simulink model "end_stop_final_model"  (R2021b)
settings: Solver=VariableStepAuto  StartTime=0.0  StopTime=20  RelTol=1e-3
libraries: fl_lib x16, nesl_utility x4, sdl_lib x1

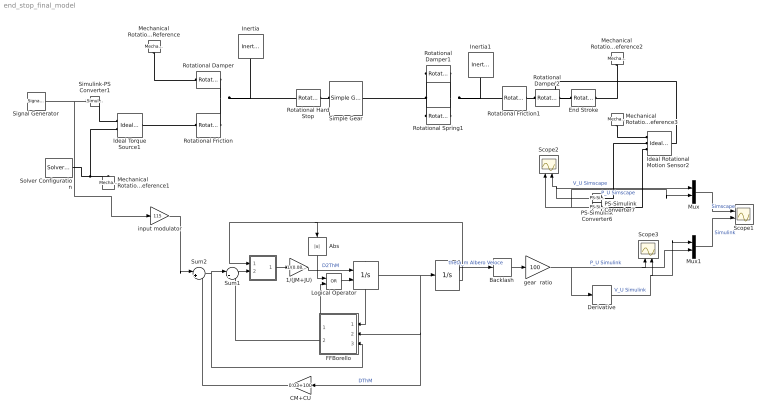
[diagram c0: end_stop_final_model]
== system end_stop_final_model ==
  " " : Integrator  ExternalReset=rising  ShowStatePort=on
  "  " : Integrator  LimitOutput=on  UpperSaturationLimit=0.1  LowerSaturationLimit=-0.1  ShowSaturationPort=on
  "                       " : Subsystem
  1/(JM+JU) : Gain  Gain=1/(0.085+50)
  Abs : Abs
  Backlash : Backlash  BacklashWidth=0.0174
  CM+CU : Gain  Gain=0.03+100
  Derivative : Derivative
  End Stroke : fl_lib/Mechanical/Rotational Elements/Rotational Hard Stop  upper_bnd=5 deg  lower_bnd=-5 deg  stiff_up=1e6 N*m/rad  stiff_low=1e6 N*m/rad  D_up=0.01 N*m/(rad/s)  D_low=0.01 N*m/(rad/s)  model=simscape.enum.hardstop.smooth  transition=0.001 rad  w_specify=off  w_priority=None  w=0 rad/s  w_nominal_specify=off  w_nominal_unit=rad/s  w_nominal_value=1  t_specify=off  t_priority=None  t=0 N*m  t_nominal_specify=off  t_nominal_unit=N*m  t_nominal_value=1  phi_specify=off  phi_priority=High  phi=0 rad  phi_nominal_specify=off  phi_nominal_unit=rad  phi_nominal_value=1
  FFBorello : Subsystem
  Ideal Rotational Motion Sensor2 : fl_lib/Mechanical/Mechanical Sensors/Ideal Rotational Motion Sensor  wrap_angle=simscape.enum.onoff.off  offset=0 rad
  Ideal Torque Source1 : fl_lib/Mechanical/Mechanical Sources/Ideal Torque Source
  Inertia : fl_lib/Mechanical/Rotational Elements/Inertia  inertia=0.085 kg*m^2  num_ports=foundation.enum.numPorts2.one  w_specify=off  w_priority=High  w=0 rad/s  w_nominal_specify=off  w_nominal_unit=rad/s  w_nominal_value=1  t_specify=off  t_priority=None  t=0 N*m  t_nominal_specify=off  t_nominal_unit=N*m  t_nominal_value=1
  Inertia1 : fl_lib/Mechanical/Rotational Elements/Inertia  inertia=50 kg*m^2  num_ports=foundation.enum.numPorts2.one  w_specify=off  w_priority=High  w=0 rad/s  w_nominal_specify=off  w_nominal_unit=rad/s  w_nominal_value=1  t_specify=off  t_priority=None  t=0 N*m  t_nominal_specify=off  t_nominal_unit=N*m  t_nominal_value=1
  Logical Operator : Logic  Operator=OR  AllPortsSameDT=off  OutDataTypeStr=boolean
  Mechanical Rotational Reference{,1..3} (4 alike) : fl_lib/Mechanical/Rotational Elements/Mechanical Rotational Reference
  Mux : Mux  Inputs=2
  Mux1 : Mux  Inputs=2
  PS-Simulink Converter6 : nesl_utility/PS-Simulink Converter  PhysicalDomain=network_engine_domain  SubClassName=ps_output  LeftPortType=input  RightPortType=output  PseudoPeriodic=off  Frequencies=[]  Unit=inherit  AffineConversion=off
  PS-Simulink Converter7 : nesl_utility/PS-Simulink Converter  PhysicalDomain=network_engine_domain  SubClassName=ps_output  LeftPortType=input  RightPortType=output  PseudoPeriodic=off  Frequencies=[]  Unit=inherit  AffineConversion=off
  Rotational Damper : fl_lib/Mechanical/Rotational Elements/Rotational Damper  D=0.03 N*m/(rad/s)  w_specify=off  w_priority=None  w=0 rad/s  w_nominal_specify=off  w_nominal_unit=rad/s  w_nominal_value=1  t_specify=off  t_priority=None  t=0 N*m  t_nominal_specify=off  t_nominal_unit=N*m  t_nominal_value=1
  Rotational Damper1 : fl_lib/Mechanical/Rotational Elements/Rotational Damper  D=50 N*m/(rad/s)  w_specify=off  w_priority=None  w=0 rad/s  w_nominal_specify=off  w_nominal_unit=rad/s  w_nominal_value=1  t_specify=off  t_priority=None  t=0 N*m  t_nominal_specify=off  t_nominal_unit=N*m  t_nominal_value=1
  Rotational Damper2 : fl_lib/Mechanical/Rotational Elements/Rotational Damper  D=100 N*m/(rad/s)  w_specify=off  w_priority=None  w=0 rad/s  w_nominal_specify=off  w_nominal_unit=rad/s  w_nominal_value=1  t_specify=off  t_priority=None  t=0 N*m  t_nominal_specify=off  t_nominal_unit=N*m  t_nominal_value=1
  Rotational Friction : fl_lib/Mechanical/Rotational Elements/Rotational Friction  brkwy_trq=5 N*m  brkwy_vel=0.1 rad/s  Col_trq=5 N*m  visc_coef=0 N*m/(rad/s)  w_specify=off  w_priority=None  w=0 rad/s  w_nominal_specify=off  w_nominal_unit=rad/s  w_nominal_value=1  t_specify=off  t_priority=None  t=0 N*m  t_nominal_specify=off  t_nominal_unit=N*m  t_nominal_value=1
  Rotational Friction1 : fl_lib/Mechanical/Rotational Elements/Rotational Friction  brkwy_trq=500 N*m  brkwy_vel=0.1 rad/s  Col_trq=500 N*m  visc_coef=0 N*m/(rad/s)  w_specify=off  w_priority=None  w=0 rad/s  w_nominal_specify=off  w_nominal_unit=rad/s  w_nominal_value=1  t_specify=off  t_priority=None  t=0 N*m  t_nominal_specify=off  t_nominal_unit=N*m  t_nominal_value=1
  Rotational Hard Stop : fl_lib/Mechanical/Rotational Elements/Rotational Hard Stop  upper_bnd=1 deg  lower_bnd=-1 deg  stiff_up=1e6 N*m/rad  stiff_low=1e6 N*m/rad  D_up=0.01 N*m/(rad/s)  D_low=0.01 N*m/(rad/s)  model=simscape.enum.hardstop.smooth  transition=0.001 rad  w_specify=off  w_priority=None  w=0 rad/s  w_nominal_specify=off  w_nominal_unit=rad/s  w_nominal_value=1  t_specify=off  t_priority=None  t=0 N*m  t_nominal_specify=off  t_nominal_unit=N*m  t_nominal_value=1  phi_specify=off  phi_priority=High  phi=0 rad  phi_nominal_specify=off  phi_nominal_unit=rad  phi_nominal_value=1
  Rotational Spring1 : fl_lib/Mechanical/Rotational Elements/Rotational Spring  spr_rate=50 N*m/rad  w_specify=off  w_priority=None  w=0 rad/s  w_nominal_specify=off  w_nominal_unit=rad/s  w_nominal_value=1  t_specify=off  t_priority=None  t=0 N*m  t_nominal_specify=off  t_nominal_unit=N*m  t_nominal_value=1  phi_specify=off  phi_priority=High  phi=0 rad  phi_nominal_specify=off  phi_nominal_unit=rad  phi_nominal_value=1
  Scope1 : Scope  NumInputPorts=2
  Scope2 : Scope  NumInputPorts=2
  Scope3 : Scope  NumInputPorts=2
  Signal Generator : SignalGenerator  Amplitude=5  Units=rad/sec
  Simple Gear : sdl_lib/Gears/Simple Gear  ratio=100  rotation_direction=sdl.enum.shaftOutputDirection.same  friction_model=sdl.enum.gear_efficiencies_load.off  T_noload=0.1 N*m  T_nom=5 N*m  efficiency_nom=0.8  efficiency=0.8  temperature_TLU=[280, 300, 320] K  load_TLU=[1, 5, 10] N*m  efficiency_TLU=[.95, .9, .85]  efficiency_TLU2=[.85, .8, .75; .95, .9, .85; .85, .8, .7]  w_thr=0.01 rad/s  pwr_thr=0.001 W  backlash_model=sdl.enum.backlashModel.Off  backlash_distance=1e-3 mm  x0=0 mm  r_base=0.1 m  hardstop_model=simscape.enum.hardstop.smooth  transition=1e-4 mm  backlash_stiffness=1e7 N/m  backlash_damping=1e6 N/(m/s)  e=0  v_tol=0.001 m/s  mu_visc=[0, 0] N*m/(rad/s)  enable_faults=simscape.enum.onoff.off  efficiency_fault=0.05  external_fault=simscape.enum.onoff.off  temporal_fault=simscape.enum.onoff.off  fault_time=5 s  fault_angles=pi / 12 rad  report_fault=simscape.enum.assert.action.none  thermal_mass=50 J/K  temperature_specify=off  temperature_priority=High  temperature=300 K  temperature_nominal_specify=off  temperature_nominal_unit=K  temperature_nominal_value=1
  Simulink-PS Converter1 : nesl_utility/Simulink-PS Converter  PhysicalDomain=network_engine_domain  SubClassName=ps_input  LeftPortType=input  RightPortType=output  PseudoPeriodic=off  Frequencies=[]  NoiseDistribution=none  NoiseParameters=[]  Unit=1  AffineConversion=off  FilteringAndDerivatives=provide  SimscapeFilterOrder=1  InputFilterTimeConstant=0.001  UdotUserProvided=0
  Solver Configuration : nesl_utility/Solver Configuration  PhysicalDomain=network_engine_domain  SubClassName=solver  LeftPortType=input  RightPortType=generic  Tones=[]  Harmonics=[]  SimulateNoise=off  Profile=off  UseLocalSampling=off  EnableSwitchedLinearOptims=on  FrequencyDomain=off  UseCCode=off  RelTol=0.001  AbsTol=1e-06  MinStep=1e-09  ToWorkspace=off  RevertToSquareIcSolve=off  NumHomotopyIterations=100  PhasorMode=off  PhasorModeNumHarmonics=1  DoDC=off  ResidualTolerance=1e-09  UseLocalSolver=off  LocalSolverChoice=NE_BACKWARD_EULER_ADVANCER  LocalSolverSampleTime=0.001  DoFixedCost=off  MaxNonlinIter=3  MaxModeIter=2  ComputeImpulses=off  ImpulseIterations=2  LinearAlgebra=auto  EquationFormulation=NE_TIME_EF  DelaysMemoryBudget=1024  AutomaticFiltering=on  FilteringTimeConstant=0.001  PartitionStorageMethod=AS_NEEDED  PartitionMemoryBudget=1024  PartitionMethod=ROBUST
  Sum1 : Sum  Inputs=|+-
  Sum2 : Sum  Inputs=|+-
  gear  ratio : Gain  Gain=100
  input modulator : Gain  Gain=115
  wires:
  PS-Simulink Converter6/1 -> Mux/1, Scope2/2  "V_U Simscape"
  PS-Simulink Converter7/1 -> Mux/2, Scope2/1  "P_U Simscape"
  Signal Generator/1 -> input modulator/1, Simulink-PS Converter1/1
  " "/State -> FFBorello/1(DThU SP)
  "  "/1 -> Backlash/1  "theta_m Albero Veloce"
  Backlash/1 -> gear  ratio/1
  1/(JM+JU)/1 -> " "/1  "D2ThM"
  Sum2/1 -> Sum1/1, FFBorello/3(Act Torque)
  " "/1 -> "  "/1, CM+CU/1, FFBorello/2(DThU)  "DThM"
  FFBorello/2(TF) -> Sum1/2
  Sum1/1 -> "                       "/2(Act ThC)
  "                       "/1(Act) -> 1/(JM+JU)/1
  "  "/2 -> Abs/1, "                       "/1(Sat Port)
  Abs/1 -> Logical Operator/1
  FFBorello/1(Reset_DXJ) -> Logical Operator/2
  Logical Operator/1 -> " "/2
  gear  ratio/1 -> Derivative/1, Mux1/2, Scope3/1  "P_U Simulink"
  CM+CU/1 -> Sum2/2
  input modulator/1 -> Sum2/1
  Derivative/1 -> Mux1/1, Scope3/2  "V_U Simulink"
  Mux/1 -> Scope1/1  "Simscape"
  Mux1/1 -> Scope1/2  "Simulink"
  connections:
  Mechanical Rotational Reference/LConn1 -- Rotational Damper/LConn1
  Ideal Torque Source1/LConn1 -- Rotational Friction/LConn1
  Rotational Friction/RConn1 -- Rotational Hard Stop/LConn1 -- Inertia/LConn1 -- Rotational Damper/RConn1
  Mechanical Rotational Reference1/LConn1 -- Solver Configuration/RConn1 -- Ideal Torque Source1/RConn2
  Rotational Hard Stop/RConn1 -- Simple Gear/LConn1
  Rotational Damper1/LConn1 -- Simple Gear/RConn1 -- Rotational Spring1/LConn1
  Rotational Damper1/RConn1 -- Rotational Friction1/LConn1 -- Inertia1/LConn1 -- Rotational Spring1/RConn1
  Mechanical Rotational Reference3/LConn1 -- Ideal Rotational Motion Sensor2/RConn1
  Ideal Rotational Motion Sensor2/RConn3 -- PS-Simulink Converter7/LConn1
  PS-Simulink Converter6/LConn1 -- Ideal Rotational Motion Sensor2/RConn2
  Simulink-PS Converter1/RConn1 -- Ideal Torque Source1/RConn1
  Rotational Damper2/RConn1 -- Rotational Friction1/RConn1
  End Stroke/LConn1 -- Ideal Rotational Motion Sensor2/LConn1 -- Rotational Damper2/LConn1
  Mechanical Rotational Reference2/LConn1 -- End Stroke/RConn1

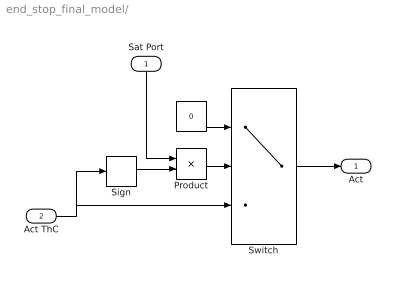
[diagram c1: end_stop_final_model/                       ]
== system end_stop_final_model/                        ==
  Sat Port : Inport
  Act ThC : Inport  Port=2
  "    " : Constant  Value=0
  Product : Product  RndMeth=Zero
  Sign : Signum
  Switch : Switch  Threshold=0.5
  Act : Outport
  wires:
  Act ThC/1 -> Switch/3, Sign/1
  Product/1 -> Switch/2
  Sign/1 -> Product/2
  "    "/1 -> Switch/1
  Switch/1 -> Act/1
  Sat Port/1 -> Product/1

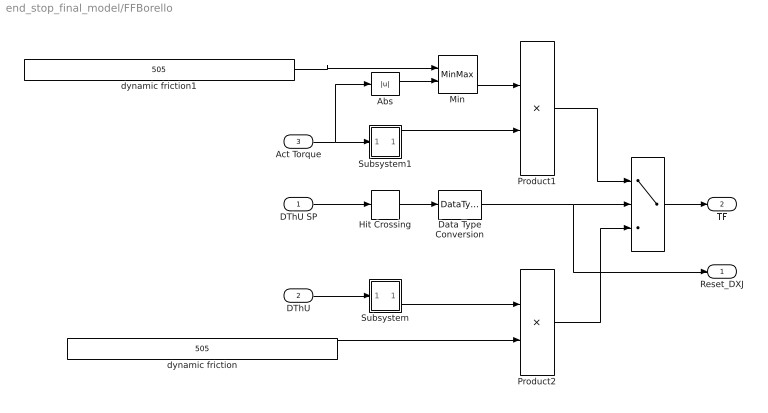
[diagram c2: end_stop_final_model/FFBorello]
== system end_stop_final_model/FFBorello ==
  DThU SP : Inport
  DThU : Inport  Port=2
  Act Torque : Inport  Port=3
  "   " : Switch  Threshold=0.5
  Abs : Abs
  Data Type Conversion : DataTypeConversion  OutDataTypeStr=double
  Hit Crossing : HitCross
  Min : MinMax  Inputs=2  InputSameDT=on  SaturateOnIntegerOverflow=on
  Product1 : Product  InputSameDT=on  RndMeth=Zero  SaturateOnIntegerOverflow=on
  Product2 : Product  InputSameDT=on  RndMeth=Zero  SaturateOnIntegerOverflow=on
  Subsystem : Subsystem
  Subsystem1 : Subsystem
  dynamic friction : Constant  Value=505
  dynamic friction1 : Constant  Value=505
  Reset_DXJ : Outport
  TF : Outport  Port=2
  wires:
  Product2/1 -> "   "/3
  DThU/1 -> Subsystem/1(In1)
  "   "/1 -> TF/1
  Product1/1 -> "   "/1
  Min/1 -> Product1/1
  Act Torque/1 -> Subsystem1/1(In1), Abs/1
  Abs/1 -> Min/2
  Hit Crossing/1 -> Data Type Conversion/1
  Subsystem/1(Out1) -> Product2/1
  Subsystem1/1(Out1) -> Product1/2
  Data Type Conversion/1 -> "   "/2, Reset_DXJ/1
  DThU SP/1 -> Hit Crossing/1
  dynamic friction1/1 -> Min/1
  dynamic friction/1 -> Product2/2

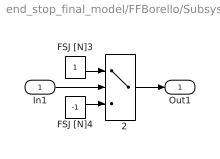
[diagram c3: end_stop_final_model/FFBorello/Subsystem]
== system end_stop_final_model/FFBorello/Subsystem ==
  In1 : Inport
  "   2" : Switch
  FSJ [N]3 : Constant
  FSJ [N]4 : Constant  Value=-1
  Out1 : Outport
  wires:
  FSJ [N]3/1 -> "   2"/1
  FSJ [N]4/1 -> "   2"/3
  In1/1 -> "   2"/2
  "   2"/1 -> Out1/1

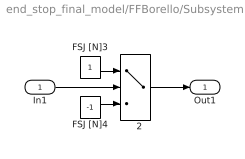
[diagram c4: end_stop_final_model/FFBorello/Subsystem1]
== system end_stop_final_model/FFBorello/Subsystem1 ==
  In1 : Inport
  "   2" : Switch
  FSJ [N]3 : Constant
  FSJ [N]4 : Constant  Value=-1
  Out1 : Outport
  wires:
  FSJ [N]3/1 -> "   2"/1
  FSJ [N]4/1 -> "   2"/3
  In1/1 -> "   2"/2
  "   2"/1 -> Out1/1
